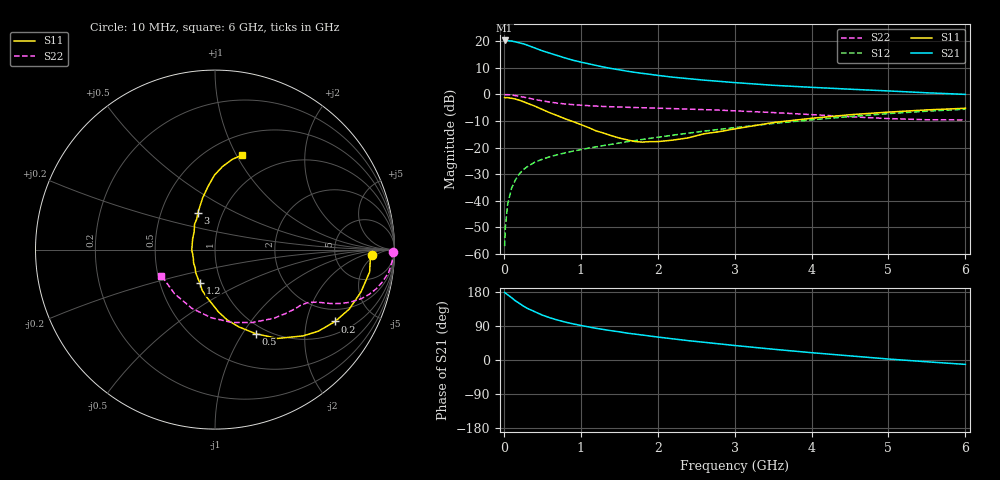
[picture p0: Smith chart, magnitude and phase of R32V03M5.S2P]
! SIEMENS Small Signal Semiconductors
! BFR181
! Si NPN RF Bipolar Junction Transistor in SOT23
! VCE = 2 V  IC = 3.5 mA
! Common Emitter S-Parameters:  May  1996
# GHz  S  MA  R  50
!  f  S11  S21  S12  S22
! GHz  MAG  ANG  MAG  ANG  MAG  ANG  MAG  ANG
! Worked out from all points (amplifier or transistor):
!   36 points, 10 MHz to 6 GHz, reference 50 ohm
!   highest |S21| = 20.3 dB at 10 MHz (marker M1)
!   |S21| within 3 dB of that: start of sweep to 418.5 MHz
!   unconditionally stable (mu >= 1): 1.25 GHz to 3.124 GHz
!   at 250 MHz: K = 0.34, MSG = 23.7 dB, |S12| = -28.4 dB
!   at 1.4 GHz: K = 1.03, MAG = 13.2 dB, |S12| = -18.7 dB
!   at 6 GHz: K = 0.86, MSG = 2.8 dB, |S12| = -5.6 dB
!   S11 on the Smith chart (normalised r, x): 10 MHz: 14, -3; 200 MHz: 1.45, -2.97; 500 MHz: 0.89, -1.15; 1.2 GHz: 0.79, -0.31; 3 GHz: 0.76, +0.33; 6 GHz: 0.70, +1.06
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0.01  0.8743 -1.8  10.35 178.5  0.0014 96.7  0.9942 -0.8
0.02  0.8668 -3.2  10.29 176.6  0.0032 83.1  0.9863 -1.6
0.05  0.8706 -8.2  10.24 172.1  0.0087 85.2  0.9894 -3.8
0.1  0.847 -16.1  10.1 164.6  0.0171 81.9  0.9767 -7.4
0.15  0.8187 -23.8  9.746 156.3  0.0246 76.3  0.9503 -10.9
0.2  0.7797 -30.9  9.353 149.7  0.0318 73.2  0.9241 -13.7
0.25  0.7342 -38.2  8.989 142.9  0.0381 70.0  0.8945 -16.2
0.3  0.6872 -44.4  8.491 136.8  0.0432 68.0  0.8619 -18.4
0.4  0.6051 -54.9  7.5 127.6  0.053 64.0  0.8056 -21.4
0.5  0.5212 -64.1  6.612 118.5  0.0604 61.5  0.7566 -23.4
0.6  0.451 -72.8  5.955 111.4  0.0675 60.0  0.7167 -24.8
0.7  0.3967 -80.3  5.364 105.3  0.0736 59.8  0.6849 -25.8
0.8  0.3466 -87.0  4.835 100.0  0.0798 58.9  0.6611 -26.5
1.1  0.2384 -107.3  3.773 87.4  0.0976 59.6  0.6145 -28.5
1.2  0.206 -114.0  3.504 83.6  0.1033 59.5  0.6034 -29.3
1.6  0.1403 -148.3  2.738 71.0  0.1289 60.8  0.5731 -32.5
2.2  0.1382 154.3  2.107 55.8  0.1716 60.4  0.5408 -39.5
3  0.2244 115.4  1.67 38.3  0.2376 56.9  0.4916 -52.1
3.5  0.2957 103.5  1.486 28.5  0.2837 53.4  0.4561 -63.0
4.5  0.4152 90.4  1.254 10.9  0.3838 43.6  0.3802 -93.2
5.5  0.5117 79.2  1.073 -4.7  0.4835 30.8  0.3335 -132.7
6  0.5493 73.9  1.002 -11.6  0.5278 23.7  0.3318 -154.1
